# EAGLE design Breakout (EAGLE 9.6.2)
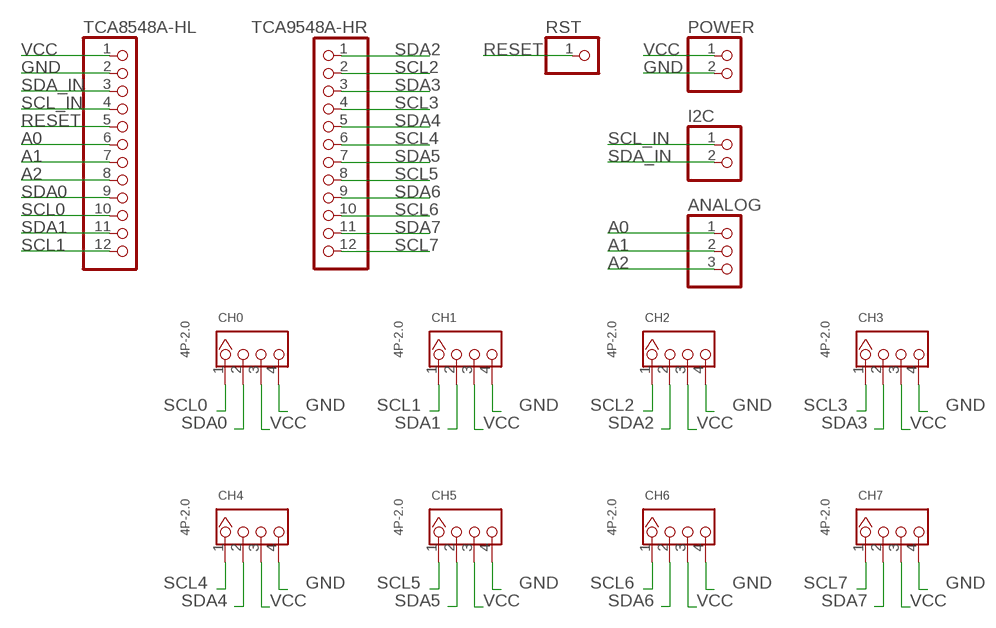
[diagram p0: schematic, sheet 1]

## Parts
ANALOG  PINHD-1X3  [1X03]
CH0  4P-2.0  GROVE-CONNECTOR-DIP(4P-2.0)  [HW4-2.0]
CH1  4P-2.0  GROVE-CONNECTOR-DIP(4P-2.0)  [HW4-2.0]
CH2  4P-2.0  GROVE-CONNECTOR-DIP(4P-2.0)  [HW4-2.0]
CH3  4P-2.0  GROVE-CONNECTOR-DIP(4P-2.0)  [HW4-2.0]
CH4  4P-2.0  GROVE-CONNECTOR-DIP(4P-2.0)  [HW4-2.0]
CH5  4P-2.0  GROVE-CONNECTOR-DIP(4P-2.0)  [HW4-2.0]
CH6  4P-2.0  GROVE-CONNECTOR-DIP(4P-2.0)  [HW4-2.0]
CH7  4P-2.0  GROVE-CONNECTOR-DIP(4P-2.0)  [HW4-2.0]
I2C  PINHD-1X2  [1X02]
POWER  PINHD-1X2  [1X02]
RST  PINHD-1X1  [1X01]
TCA8548A-HL  PINHD-1X12  [1X12]
TCA9548A-HR  PINHD-1X12  [1X12]

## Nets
A0 [Workshop]: ANALOG.1 TCA8548A-HL.6
A1 [Workshop]: ANALOG.2 TCA8548A-HL.7
A2 [Workshop]: ANALOG.3 TCA8548A-HL.8
GND [Workshop]: CH0.4 CH1.4 CH2.4 CH3.4 CH4.4 CH5.4 CH6.4 CH7.4 POWER.2 TCA8548A-HL.2
RESET [Workshop]: RST.1 TCA8548A-HL.5
SCL0 [Workshop]: CH0.1 TCA8548A-HL.10
SCL1 [Workshop]: CH1.1 TCA8548A-HL.12
SCL2 [Workshop]: CH2.1 TCA9548A-HR.2
SCL3 [Workshop]: CH3.1 TCA9548A-HR.4
SCL4 [Workshop]: CH4.1 TCA9548A-HR.6
SCL5 [Workshop]: CH5.1 TCA9548A-HR.8
SCL6 [Workshop]: CH6.1 TCA9548A-HR.10
SCL7 [Workshop]: CH7.1 TCA9548A-HR.12
SCL_IN [Workshop]: I2C.1 TCA8548A-HL.4
SDA0 [Workshop]: CH0.2 TCA8548A-HL.9
SDA1 [Workshop]: CH1.2 TCA8548A-HL.11
SDA2 [Workshop]: CH2.2 TCA9548A-HR.1
SDA3 [Workshop]: CH3.2 TCA9548A-HR.3
SDA4 [Workshop]: CH4.2 TCA9548A-HR.5
SDA5 [Workshop]: CH5.2 TCA9548A-HR.7
SDA6 [Workshop]: CH6.2 TCA9548A-HR.9
SDA7 [Workshop]: CH7.2 TCA9548A-HR.11
SDA_IN [Workshop]: I2C.2 TCA8548A-HL.3
VCC [Workshop]: CH0.3 CH1.3 CH2.3 CH3.3 CH4.3 CH5.3 CH6.3 CH7.3 POWER.1 TCA8548A-HL.1

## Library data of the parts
ANALOG = pinhead:PINHD-1X3: PIN HEADER
CH0 CH1-CH7 = OPL_Connector:GROVE-CONNECTOR-DIP(4P-2.0): 320110033
I2C POWER = pinhead:PINHD-1X2: PIN HEADER
RST = pinhead:PINHD-1X1: PIN HEADER
TCA8548A-HL TCA9548A-HR = pinhead:PINHD-1X12: PIN HEADER

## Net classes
1 Workshop: width 0.4 mm, clearance 0.2 mm

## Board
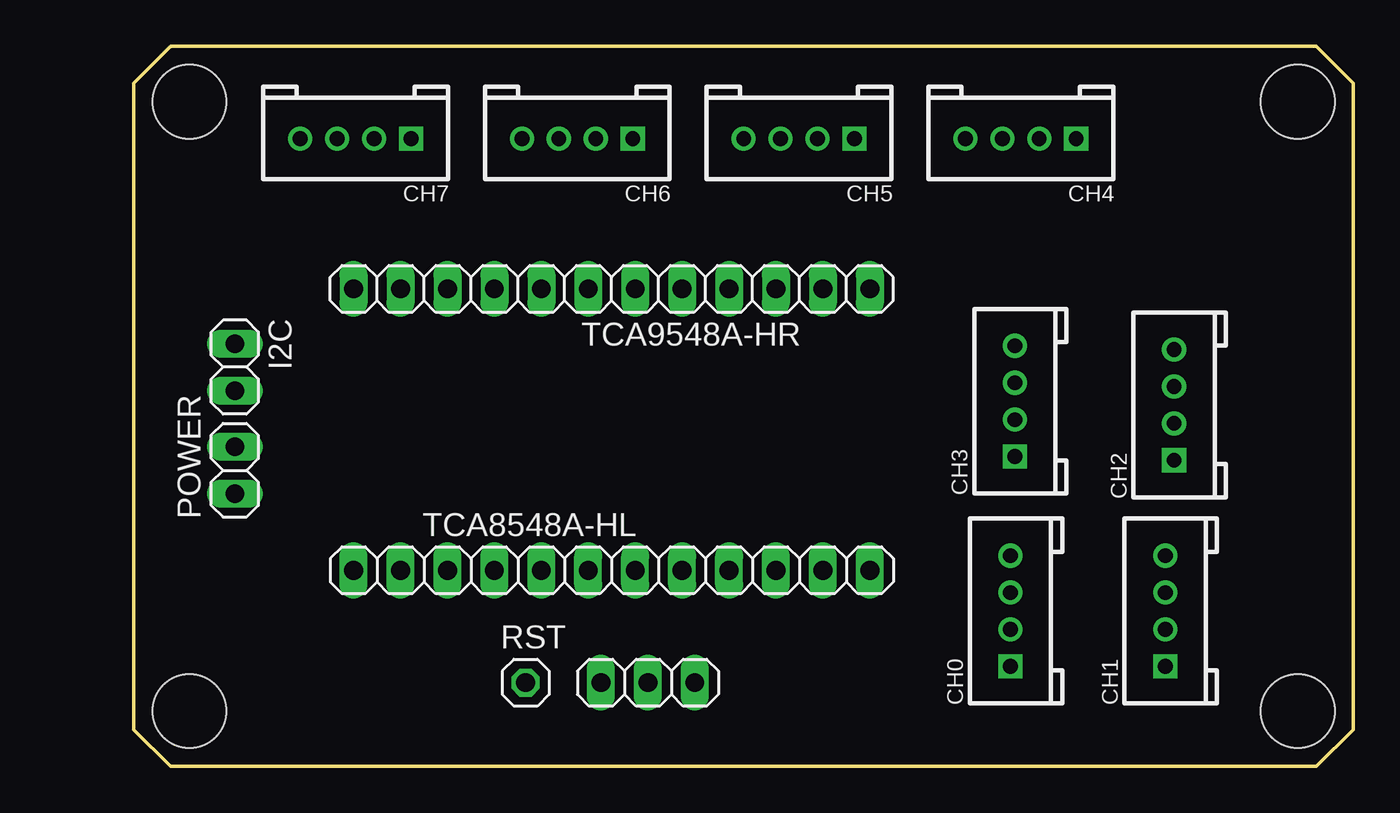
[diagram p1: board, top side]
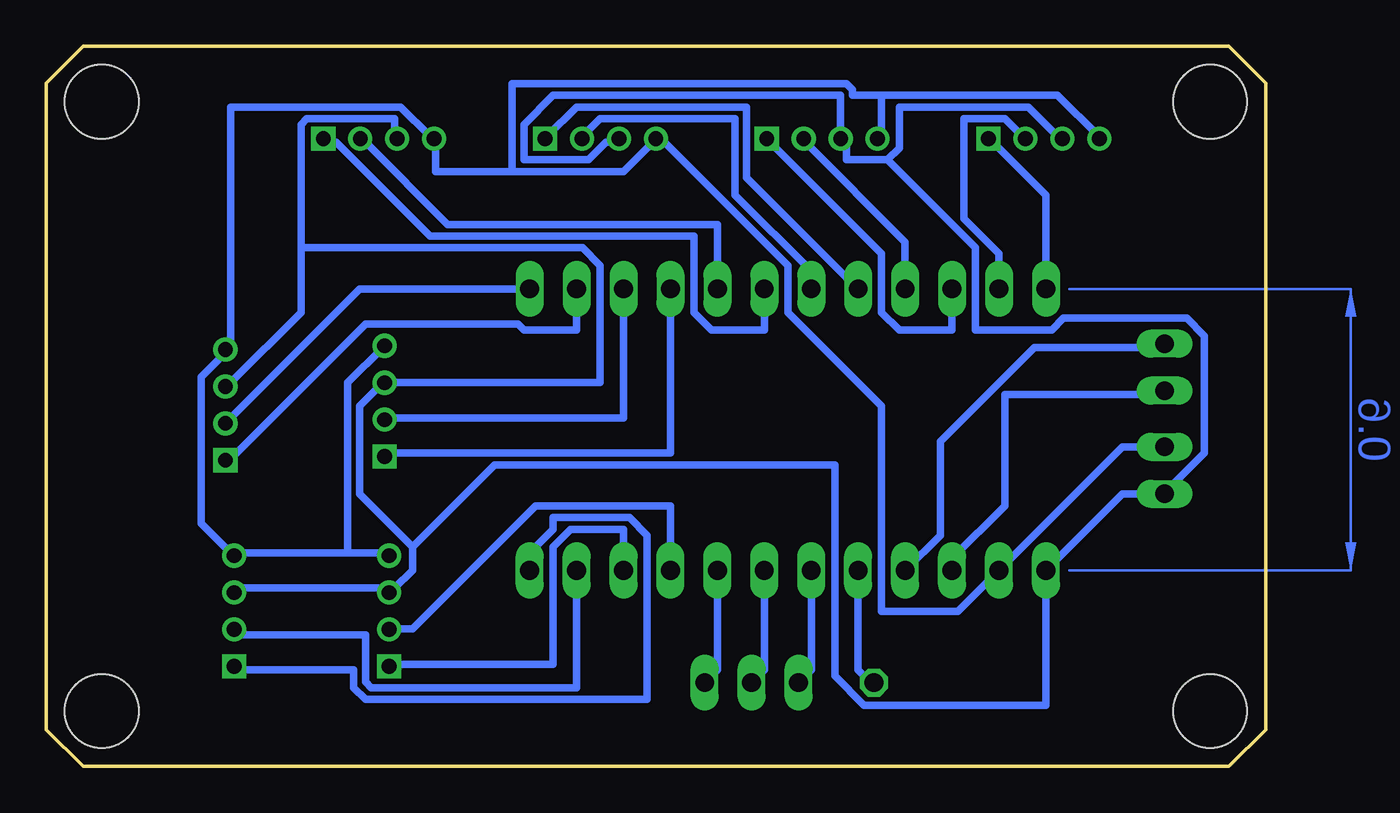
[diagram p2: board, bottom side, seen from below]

Size 66 x 39 mm. Coordinates in mm from the lower left corner, seen from the top.
Outline: 0,2 0,37 2,39 64,39 66,37 66,2 64,0 2,0 0,2
Copper layers (1*16): Top 0.035mm / dielectric 1.5mm / Bottom 0.035mm
Design rules "default": minimum track width 6mil, minimum drill 0.35mm, track to track 6mil, track to pad 6mil, pad to pad 6mil, via to via 6mil, smd to smd 6mil, copper to edge 40mil, drill to drill 6mil, minimum pad ring 10mil, minimum via ring 8mil, stop-mask expansion 4mil, vias tented up to drill 0mil, thermal gap 10mil
Holes 4 mm at 3,3 63,3 63,36 3,36

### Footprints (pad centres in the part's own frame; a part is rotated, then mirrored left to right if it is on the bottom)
1X03 = drill 1.016 long: 1 -2.54,0; 2 0,0; 3 2.54,0
HW4-2.0 = drill 0.8 pad 1.27 square: 1 -3,0 | drill 0.8 pad 1.27: 2 -1,0; 3 1,0; 4 3,0
1X02 = drill 1.016 long: 1 -1.27,0; 2 1.27,0
1X01 = drill 1.016 octagon: 1 0,0
1X12 = drill 1.016 long: 1 -13.97,0; 2 -11.43,0; 3 -8.89,0; 4 -6.35,0; 5 -3.81,0; 6 -1.27,0; 7 1.27,0; 8 3.81,0; 9 6.35,0; 10 8.89,0; 11 11.43,0; 12 13.97,0

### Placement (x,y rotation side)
ANALOG  27.82,4.54 0 top
CH0  47.44,8.42 90 top
CH1  55.82,8.42 90 top
CH2  56.3,19.58 90 top
CH3  47.68,19.78 90 top
CH4  48,34 180 top
CH5  36,34 180 top
CH6  24,34 180 top
CH7  12,34 180 top
I2C  5.46,21.62 270 top
POWER  5.46,16.04 90 top
RST  21.2,4.54 0 top
TCA8548A-HL  25.86,10.62 0 top
TCA9548A-HR  25.86,25.86 180 top

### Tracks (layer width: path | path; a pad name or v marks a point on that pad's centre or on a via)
A0
  Bottom 0.4: TCA8548A-HL.6 24.59,5.22 25.23,4.59 ANALOG.1
A1
  Bottom 0.4: TCA8548A-HL.7 27.13,5.22 27.77,4.59 ANALOG.2
A2
  Bottom 0.4: TCA8548A-HL.8 29.67,5.22 30.3,4.59 ANALOG.3
GND
  Bottom 0.4: POWER.2 5.54,17.29 7.76,17.29 TCA8548A-HL.2 16.65,8.4 20.78,8.4 20.78,19.51 25.86,24.59 25.86,27.13 32.84,34.11 CH5.4 33.16,33.8 34.75,32.21 40.78,32.21 | 20.78,36.34 11.26,36.34 9.03,34.11 CH7.4 | 20.78,36.34 20.78,34.11 CH6.4 | 40.78,32.21 44.91,32.21 44.91,33.8 CH4.4 45.23,34.11 46.81,35.7 56.02,35.7 56.02,22.68 CH2.4 56.34,22.37 57.61,21.1 57.61,13.16 56.02,11.57 CH1.4 55.7,11.57 49.67,11.57 | 49.67,11.57 47.45,11.57 CH0.4 | 49.67,11.57 49.67,20.78 47.77,22.68 CH3.4 | 20.78,36.34 22.37,36.34 22.37,36.66 22.68,36.97 40.78,36.97 40.78,32.21
RESET
  Bottom 0.4: TCA8548A-HL.5 22.05,5.22 21.41,4.59 RST.1
SCL0
  Bottom 0.4: TCA8548A-HL.10 34.75,12.84 37.61,12.84 38.56,11.89 38.56,5.54 47.13,5.54 CH0.1
SCL1
  Bottom 0.4: TCA8548A-HL.12 39.83,11.57 38.56,12.84 38.56,13.48 34.43,13.48 33.48,12.53 33.48,3.63 48.72,3.63 49.35,4.27 49.35,5.22 55.7,5.22 CH1.1
SCL2
  Bottom 0.4: TCA9548A-HR.2 37.29,23.64 40.15,23.64 40.47,23.95 48.72,23.95 56.02,16.65 CH2.1
SCL3
  Bottom 0.4: TCA9548A-HR.4 32.21,16.97 47.45,16.97 CH3.1
SCL4
  Bottom 0.4: TCA9548A-HR.6 27.13,23.64 29.99,23.64 30.94,24.59 30.94,28.72 45.23,28.72 50.31,33.8 50.94,33.8 CH4.1
SCL5
  Bottom 0.4: TCA9548A-HR.8 28.08,31.89 28.08,35.7 37.29,35.7 38.88,34.11 CH5.1
SCL6
  Bottom 0.4: TCA9548A-HR.10 16.97,23.64 19.83,23.64 20.78,24.59 20.78,27.77 26.81,33.8 CH6.1
SCL7
  Bottom 0.4: TCA9548A-HR.12 11.89,30.94 14.75,33.8 CH7.1
SCL_IN
  Bottom 0.4: TCA8548A-HL.4 17.61,12.53 17.61,17.61 12.53,22.68 5.54,22.68 I2C.1
SDA0
  Bottom 0.4: TCA8548A-HL.9 32.21,14.11 39.51,14.11 46.18,7.45 47.13,7.45 CH0.2
SDA1
  Bottom 0.4: TCA8548A-HL.11 37.29,4.27 48.4,4.27 48.72,4.59 48.72,7.13 55.7,7.13 CH1.2
SDA2
  Bottom 0.4: TCA9548A-HR.1 49.04,25.86 56.02,18.88 CH2.2
SDA3
  Bottom 0.4: TCA9548A-HR.3 34.75,18.88 47.45,18.88 CH3.2
SDA4
  Bottom 0.4: TCA9548A-HR.5 29.67,29.35 44.27,29.35 48.72,33.8 CH4.2
SDA5
  Bottom 0.4: TCA9548A-HR.7 24.59,26.81 28.72,30.94 28.72,35.07 36.02,35.07 36.97,34.11 CH5.2
SDA6
  Bottom 0.4: TCA9548A-HR.9 19.51,28.4 24.91,33.8 CH6.2
SDA7
  Bottom 0.4: TCA9548A-HR.11 14.43,27.77 16.34,29.67 16.34,35.07 14.11,35.07 13.16,34.11 CH7.2
SDA_IN
  Bottom 0.4: TCA8548A-HL.3 16.97,11.26 14.11,14.11 14.11,20.14 5.54,20.14 I2C.2
VCC
  Bottom 0.4: CH1.3 55.7,9.67 47.45,9.67 CH0.3 47.13,9.67 46.18,10.62 46.18,11.89 | 46.18,11.89 49.04,14.75 49.04,19.51 47.77,20.78 CH3.3 36.02,20.78 36.02,27.13 36.97,28.08 52.21,28.08 | 52.21,28.08 52.21,34.75 51.9,35.07 47.13,35.07 47.13,34.11 CH4.3 | 52.21,28.08 52.21,24.59 56.02,20.78 CH2.3 | 20.46,32.84 19.83,33.48 19.83,35.7 12.84,35.7 11.26,34.11 CH7.3 | 20.46,32.84 22.68,32.84 22.68,33.8 CH6.3 23,34.11 23,36.34 38.56,36.34 40.15,34.75 40.15,32.84 36.66,32.84 35.7,33.8 35.07,33.8 CH5.3 | 20.46,32.84 15.7,28.08 15.7,23.64 11.57,23.64 10.94,24.27 4.27,24.27 3.32,23.32 3.32,16.97 5.22,15.06 POWER.1 5.54,14.75 7.76,14.75 TCA8548A-HL.1 11.89,3.32 21.73,3.32 23.32,4.91 23.32,16.34 41.73,16.34 46.18,11.89
(copper drawn outside any net)
  shapes: Bottom area x1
